[IBIS Ver]   4.1
[File Name]   tms570ls31x_21x_revc_pge_b.ibs
[File Rev]   1.0
[Date]   Tue Sep 17 07:21:23 2013
[Source]   Texas Instruments, Inc.
[Notes]   Revision History:
   1.0: initial release, 09/17/2013
   THIS IS RELEASE 1.0,THE CONTENTS ARE SUBJECT TO
   CHANGE WITHOUT PRIOR NOTICE,IF NECESSARY.
[Disclaimer] Please be aware that in the absence of a written agreement
   Texas Instruments(TI) assumes no liability for:
   (1) The accuracy of the IBIS models provided to your company
   (2) The proper functioning of these Models in your design
   or for any resulting applications;or
   (3) Infringement of patents,copyrights or intellectual
   property rights resulting from your use of these models.
   TI provides IBIS Models as a service to our customers and
   therefore reserves the right to limit distribution of the
   Models.
[Copyright]   Property of Texas Instruments Incorporated.
   Unauthorised reproduction and/or distribution is strictly.
   prohibited.
   This product is protected under copyright law and trade
   secret law as an unpublished work.
   Created 2013,(C) Copyright 2013-2014,
   Texas Instruments Incorporated., All Rights Reserved.
   These commodities are under the U.S. Government
   distribution license control.As such,they are not to be
   re-exported without the prior approval of the
   U.S. Department of Commerce.
[Component]   TMS570LS31x/21x_REVC_PGE_B
[Manufacturer]   Texas Instruments
[Package]
 | variable   typ   min   max
R_pkg   179.763m   7.91949m   216.493m
L_pkg   7.02661nH   2.0891nH   7.71072nH
C_pkg   0.955318pF   0.771641pF   6.68767pF
[Pin]	signal_name	model_name	R_pin	L_pin	C_pin
1	FRAYTX2	OQ0112FT	201.684m	7.04026nH	0.937901pF
2	FRAYRX2	IQ0442FT_40P60P	200.916m	7.42774nH	1.06436pF
3	MIBSPI3NCS[3]	BQ0210FT	198.584m	7.59867nH	1.05403pF
4	MIBSPI3NCS[2]	BQ0210FT	195.911m	7.63854nH	1.03198pF
5	FRAYTXEN2	OQ0112FT	195.321m	7.65814nH	1.00344pF
6	NHET1[11]	BQ0210FT	195.924m	7.67408nH	0.970612pF
|7	FLTP1	BAFTHRU15VFT	196.228m	7.64822nH	0.953678pF
|8	FLTP2	BAFTHRU8VFT	196.899m	7.58856nH	0.936175pF
9	GIOA[2]	BQ0215FT	200.797m	7.59854nH	0.910668pF
|10	VCCIO	VDDS33TF1_60UM	204.628m	7.57516nH	0.908233pF
|11	VSS	VSS00T2_60UM	203.393m	7.46268nH	0.896311pF
12	CAN3RX	BQ0210FT	204.531m	7.41325nH	0.865383pF
13	CAN3TX	BQ0210FT	212.37m	7.50397nH	0.859888pF
14	GIOA[5]	BQ0210FT	213.785m	7.48678nH	0.855034pF
15	NHET1[22]	BQ0215FT	213.017m	7.33523nH	0.854962pF
16	GIOA[6]	BQ0210FT	211.155m	7.25549nH	0.844253pF
|17	VCC	VDD12T1_100UM	120.798m	6.70564nH	0.867718pF
|18	OSCIN	IOSCHF33FTHY_NI	214.999m	7.2584nH	0.815084pF
|19	KELVIN_GND	VSS00T2_60UM	213.472m	7.23357nH	0.828091pF
|20	OSCOUT	OOSCHF33FT	209.627m	7.16687nH	0.835423pF
|21	VSS	VSS00T2_60UM	206.908m	7.15454nH	0.828833pF
22	GIOA[7]	BQ0210FT	207.016m	7.17268nH	0.825821pF
23	NHET1[01]	BQ0215FT	205.654m	7.15804nH	0.858767pF
24	NHET1[03]	BQ0215FT	202.592m	7.0987nH	0.878742pF
25	NHET1[0]	BQ0215FT	201.398m	7.17984nH	0.889476pF
|26	VCCIO	VDDS33TF1_60UM	116.258m	6.76964nH	0.963387pF
|27	VSS	VSS00T2_60UM	198.771m	7.34545nH	0.926279pF
|28	VSS	VSS00T2_60UM	198.014m	7.38253nH	0.949683pF
|29	VCC	VDD12T1_100UM	116.537m	6.9325nH	1.02223pF
30	NHET1[02]	BQ0215FT	198.729m	7.45545nH	0.966564pF
31	NHET1[05]	BQ0215FT	198.508m	7.51746nH	0.97276pF
32	MIBSPI5NCS[0]	BQ0210FT	198.713m	7.58776nH	1.00435pF
33	NHET1[07]	BQ0215FT	198.824m	7.63516nH	1.03075pF
34	TEST	BQ0213FT	202.469m	7.64935nH	1.04432pF
35	NHET1[09]	BQ0215FT	198.884m	7.46111nH	1.04914pF
36	NHET1[04]	BQ0210FT	201.493m	7.12235nH	0.932251pF
37	MIBSPI3NCS[1]	BQ0215FT	189.818m	6.90291nH	0.941411pF
38	NHET1[06]	BQ0210FT	181.261m	7.14802nH	1.05899pF
39	NHET1[13]	BQ0210FT	181.614m	7.41222nH	1.03625pF
40	MIBSPI1NCS[2]	BQ0215FT	174.499m	7.33051nH	1.01977pF
41	NHET1[15]	BQ0210FT	168.874m	7.24167nH	0.998916pF
|42	VCCIO	VDDS33TF1_60UM	164.766m	7.11249nH	0.963348pF
|43	VSS	VSS00T2_60UM	161.622m	6.97546nH	0.946437pF
|44	VSS	VSS00T2_60UM	159.787m	6.88564nH	0.937131pF
|45	VCC	VDD12T1_100UM	75.8295m	6.24953nH	0.974078pF
46	nPORRST	IQ0087FT	162.699m	6.8213nH	0.87771pF
|47	VSS	VSS00T2_60UM	161.89m	6.69562nH	0.870364pF
|48	VCC	VDD12T1_100UM	97.1908m	6.22797nH	0.900575pF
|49	VCC	VDD12T1_100UM	96.9924m	6.13153nH	0.88635pF
|50	VSS	VSS00T2_60UM	164.702m	6.51157nH	0.826317pF
51	MIBSPI3SOMI	BQ0211FT	166.102m	6.43655nH	0.804429pF
52	MIBSPI3SIMO	BQ0211FT	167.111m	6.3794nH	0.795778pF
53	MIBSPI3CLK	BQ0211FT	169.065m	6.34914nH	0.786551pF
54	MIBSPI3NENA	BQ0210FT	171.864m	6.3567nH	0.784271pF
55	MIBSPI3NCS[0]	BQ0210FT	174.472m	6.49861nH	0.788938pF
|56	VSS	VSS00T2_60UM	174.866m	6.48726nH	0.784451pF
|57	VCC	VDD12T1_100UM	76.8843m	5.8157nH	0.84495pF
|58	AD1IN[16]_AD2IN[0]	IQ0444FT5	167.871m	6.39938nH	0.7931pF
|59	AD1IN[17]_AD2IN[01]	IQ0444FT5	165.448m	6.40474nH	0.816553pF
|60	AD1IN[0]	IQ0078FT5	163.468m	6.43102nH	0.836345pF
|61	AD1IN[07]	IQ0078FT5	162.275m	6.47546nH	0.851244pF
|62	AD1IN[18]_AD2IN[02]	IQ0444FT5	161.555m	6.56596nH	0.859126pF
|63	AD1IN[19]_AD2IN[03]	IQ0444FT5	161.432m	6.67329nH	0.869256pF
|64	AD1IN[20]_AD2IN[04]	IQ0444FT5	161.381m	6.70182nH	0.90007pF
|65	AD1IN[21]_AD2IN[05]	IQ0444FT5	161.995m	6.77747nH	0.921382pF
|66	ADREFHI	BAFTHRU50FT	162.542m	6.90485nH	0.933116pF
|67	ADREFLO	BAFTHRU50FT	164.993m	7.01966nH	0.953953pF
|68	VSSAD	VSSA00T2_100UM	167.891m	7.07177nH	0.987652pF
|69	VCCAD	VDDA50TF2	171.939m	7.12571nH	1.0092pF
|70	AD1IN[09]_AD2IN[09]	IQ0444FT5	176.774m	7.19031nH	1.02717pF
|71	AD1IN[01]	IQ0078FT5	182.269m	7.07161nH	1.05417pF
|72	AD1IN[10]_AD2IN[10]	IQ0444FT5	188.41m	6.88307nH	0.930632pF
|73	AD1IN[02]	IQ0078FT5	199.512m	7.07604nH	0.937836pF
|74	AD1IN[03]	IQ0078FT5	196.43m	7.45714nH	1.06151pF
|75	AD1IN[11]_AD2IN[11]	IQ0444FT5	195.408m	7.65087nH	1.04087pF
|76	AD1IN[04]	IQ0078FT5	194.285m	7.71072nH	1.02379pF
|77	AD1IN[12]_AD2IN[12]	IQ0444FT5	194.295m	7.68045nH	1.00758pF
|78	AD1IN[05]	IQ0078FT5	195.169m	7.65467nH	0.97891pF
|79	AD1IN[13]_AD2IN[13]	IQ0444FT5	195.708m	7.58317nH	0.966122pF
|80	AD1IN[06]	IQ0078FT5	198.156m	7.53735nH	0.95599pF
|81	AD1IN[22]_AD2IN[06]	IQ0444FT5	199.148m	7.54285nH	0.92948pF
|82	AD1IN[14]_AD2IN[14]	IQ0444FT5	201.452m	7.53971nH	0.90262pF
|83	AD1IN[08]_AD2IN[08]	IQ0444FT5	204.034m	7.4573nH	0.891661pF
|84	AD1IN[23]_AD2IN[07]	IQ0444FT5	205.119m	7.4742nH	0.883899pF
|85	AD1IN[15]_AD2IN[15]	IQ0444FT5	206.638m	7.35868nH	0.864379pF
86	AD1EVT	BQ0210FT	205.68m	7.30192nH	0.836559pF
|87	VCC	VDD12T1_100UM	88.0539m	6.42383nH	0.922308pF
|88	VSS	VSS00T2_60UM	205.44m	7.16036nH	0.846531pF
89	CAN1TX	BQ0210FT	207.947m	7.16054nH	0.837647pF
90	CAN1RX	BQ0210FT	211.017m	7.16768nH	0.82523pF
91	NHET1[24]	BQ0210FT	212.306m	7.15051nH	0.826669pF
92	NHET1[26]	BQ0210FT	213.491m	7.22891nH	0.844168pF
93	MIBSPI1SIMO	BQ0211FT	215.474m	7.31019nH	0.845545pF
94	MIBSPI1SOMI	BQ0211FT	214.506m	7.3229nH	0.83827pF
95	MIBSPI1CLK	BQ0211FT	213.809m	7.40217nH	0.868381pF
96	MIBSPI1NENA	BQ0210FT	216.493m	7.50172nH	0.884186pF
97	MIBSPI5NENA	BQ0210FT	210.996m	7.42558nH	0.870334pF
98	MIBSPI5SOMI[0]	BQ0212FT	207.913m	7.31239nH	0.881672pF
99	MIBSPI5SIMO[0]	BQ0212FT	206.103m	7.33234nH	0.903194pF
100	MIBSPI5CLK	BQ0212FT	206.76m	7.43485nH	0.929874pF
|101	VCC	VDD12T1_100UM	199.781m	7.44261nH	0.938448pF
|102	VSS	VSS00T2_60UM	199.165m	7.56763nH	0.948344pF
|103	VSS	VSS00T2_60UM	197.046m	7.56124nH	0.976045pF
|104	VCCIO	VDDS33TF1_60UM	197.927m	7.57833nH	1.00913pF
105	MIBSPI1NCS[0]	BQ0215FT	196.658m	7.59451nH	1.02357pF
106	NHET1[08]	BQ0215FT	199.189m	7.59472nH	1.0449pF
107	NHET1[28]	BQ0215FT	198.581m	7.39713nH	1.04993pF
108	TMS	BQ0192FT	199.808m	7.05039nH	0.92717pF
109	nTRST	IQ0087FT	189.351m	6.93314nH	0.941519pF
110	TDI	BQ0192FT	180.833m	7.18053nH	1.06865pF
111	TDO	BQ0192FT	174.6m	7.30146nH	1.04099pF
112	TCK	IQ0079FT	168.129m	7.20332nH	1.0074pF
113	RTCK	OQ0112FT	164.996m	7.10969nH	0.971868pF
|114	VCC	VDD12T1_100UM	183.392m	7.38873nH	0.965351pF
|115	VSS	VSS00T2_60UM	178.077m	7.27224nH	0.953382pF
116	nRST	BQ0414FT	176.952m	7.2215nH	0.937805pF
117	nERROR	BQ0212FT	174.143m	7.11039nH	0.912062pF
118	NHET1[10]	BQ0215FT	174.219m	6.97097nH	0.889169pF
119	ECLK	BQ0215FT	170.748m	6.83875nH	0.875206pF
|120	VCCIO	VDDS33TF1_60UM	169.236m	6.73321nH	0.861787pF
|121	VSS	VSS00T2_60UM	166.709m	6.63449nH	0.840897pF
|122	VSS	VSS00T2_60UM	169.916m	6.72922nH	0.81904pF
|123	VCC	VDD12T1_100UM	99.72m	6.24773nH	0.842834pF
124	NHET1[12]	BQ0210FT	174.231m	6.61843nH	0.792641pF
125	NHET1[14]	BQ0215FT	173.472m	6.52561nH	0.783236pF
126	FRAYRX1	IQ0442FT_40P60P	173.246m	6.47199nH	0.771641pF
127	NHET1[30]	BQ0215FT	173.833m	6.46115nH	0.771688pF
128	CAN2TX	BQ0210FT	170.744m	6.41525nH	0.773058pF
129	CAN2RX	BQ0210FT	173.471m	6.45308nH	0.801657pF
130	MIBSPI1NCS[1]	BQ0215FT	169.083m	6.38503nH	0.815094pF
131	LINRX	BQ0210FT	166.559m	6.35471nH	0.824822pF
132	LINTX	BQ0210FT	163.671m	6.38226nH	0.836538pF
133	FRAYTX1	OQ0112FT	162.88m	6.42987nH	0.839891pF
|134	VCCP	VDDFT33TF	97.1337m	6.10946nH	0.895144pF
|135	VSS	VSS00T2_60UM	160.618m	6.63246nH	0.877099pF
|136	VCCIO	VDDS33TF1_60UM	159.375m	6.64065nH	0.908634pF
|137	VCC	VDD12T1_100UM	159.405m	6.687nH	0.928827pF
|138	VSS	VSS00T2_60UM	160.655m	6.80407nH	0.940362pF
139	NHET1[16]	BQ0210FT	163.282m	6.89936nH	0.962829pF
140	NHET1[18]	BQ0210FT	166.657m	6.95055nH	0.998875pF
141	NHET1[20]	BQ0210FT	171.862m	7.00459nH	1.01785pF
142	FRAYTXEN1	OQ0112FT	178.736m	7.09847nH	1.03593pF
|143	VCC	VDD12T1_100UM	181.802m	7.01727nH	1.05637pF
|144	VSS	VSS00T2_60UM	189.553m	6.84899nH	0.943956pF
[Model Selector] BQ0192FT
BQ0192FT_PZ_3P3  Cell operated at 3.3(nom)
|BQ0192FT_PZ_3P3; PUPD_OFF
BQ0192FT_PU_3P3  Cell operated at 3.3(nom)
|BQ0192FT_PU_3P3; PULLUP_ON
BQ0192FT_PD_3P3  Cell operated at 3.3(nom)
|BQ0192FT_PD_3P3; PULLDOWN_ON
[Model Selector] BQ0210FT
BQ0210FT_PZ_3P3  Cell operated at 3.3(nom)
|BQ0210FT_PZ_3P3; PUPD_OFF
BQ0210FT_PU_3P3  Cell operated at 3.3(nom)
|BQ0210FT_PU_3P3; PULLUP_ON
BQ0210FT_PD_3P3  Cell operated at 3.3(nom)
|BQ0210FT_PD_3P3; PULLDOWN_ON
[Model Selector] BQ0211FT
BQ0211FT_PZ_3P3  Cell operated at 3.3(nom)
|BQ0211FT_PZ_3P3; PUPD_OFF
BQ0211FT_PU_3P3  Cell operated at 3.3(nom)
|BQ0211FT_PU_3P3; PULLUP_ON
BQ0211FT_PD_3P3  Cell operated at 3.3(nom)
|BQ0211FT_PD_3P3; PULLDOWN_ON
[Model Selector] BQ0212FT
BQ0212FT_PZ_3P3  Cell operated at 3.3(nom)
|BQ0212FT_PZ_3P3; PUPD_OFF
BQ0212FT_PU_3P3  Cell operated at 3.3(nom)
|BQ0212FT_PU_3P3; PULLUP_ON
BQ0212FT_PD_3P3  Cell operated at 3.3(nom)
|BQ0212FT_PD_3P3; PULLDOWN_ON
[Model Selector] BQ0213FT
BQ0213FT_PZ_3P3  Cell operated at 3.3(nom)
|BQ0213FT_PZ_3P3; PULLDOWN_OFF
BQ0213FT_PD_3P3  Cell operated at 3.3(nom)
|BQ0213FT_PD_3P3; PULLDOWN_ON
[Model Selector] BQ0215FT
BQ0215FT_PZ_3P3  Cell operated at 3.3(nom)
|BQ0215FT_PZ_3P3; PUPD_OFF
BQ0215FT_PU_3P3  Cell operated at 3.3(nom)
|BQ0215FT_PU_3P3; PULLUP_ON
BQ0215FT_PD_3P3  Cell operated at 3.3(nom)
|BQ0215FT_PD_3P3; PULLDOWN_ON
[Model Selector] BQ0414FT
BQ0414FT_PZ_3P3  Cell operated at 3.3(nom)
|BQ0414FT_PZ_3P3; PUPD_OFF
BQ0414FT_PU_3P3  Cell operated at 3.3(nom)
|BQ0414FT_PU_3P3; PULLUP_ON
BQ0414FT_PD_3P3  Cell operated at 3.3(nom)
|BQ0414FT_PD_3P3; PULLDOWN_ON
[Model Selector] IQ0079FT
IQ0079FT_PZ_3P3  Cell operated at 3.3(nom)
|IQ0079FT_PZ_3P3; PUPD_OFF
IQ0079FT_PU_3P3  Cell operated at 3.3(nom)
|IQ0079FT_PU_3P3; PULLUP_ON
IQ0079FT_PD_3P3  Cell operated at 3.3(nom)
|IQ0079FT_PD_3P3; PULLDOWN_ON
[Model Selector] IQ0087FT
IQ0087FT_PZ_3P3  Cell operated at 3.3(nom)
|IQ0087FT_PZ_3P3; PULLDOWN_OFF
IQ0087FT_PD_3P3  Cell operated at 3.3(nom)
|IQ0087FT_PD_3P3; PULLDOWN_ON
[Model Selector] IQ0442FT_40P60P
0442FT_40P60P_PZ_3P3  Cell operated at 3.3(nom)
|IQ0442FT_40P60P_PZ_3P3; PUPD_OFF
2FT_40P60P_PU_3P3  Cell operated at 3.3(nom)
|IQ0442FT_40P60P_PU_3P3; PULLUP_ON
2FT_40P60P_PD_3P3  Cell operated at 3.3(nom)
| Models and submodels in the file (29): BQ0192FT_PZ_3P3 (I/O), BQ0192FT_PU_3P3 (I/O), BQ0192FT_PD_3P3 (I/O), BQ0210FT_PZ_3P3 (I/O), BQ0210FT_PU_3P3 (I/O), BQ0210FT_PD_3P3 (I/O), BQ0211FT_PZ_3P3 (I/O), BQ0211FT_PU_3P3 (I/O), BQ0211FT_PD_3P3 (I/O), BQ0212FT_PZ_3P3 (I/O), BQ0212FT_PU_3P3 (I/O), BQ0212FT_PD_3P3 (I/O), BQ0213FT_PZ_3P3 (I/O), BQ0213FT_PD_3P3 (I/O), BQ0215FT_PZ_3P3 (I/O), BQ0215FT_PU_3P3 (I/O), BQ0215FT_PD_3P3 (I/O), BQ0414FT_PZ_3P3 (I/O), BQ0414FT_PU_3P3 (I/O), BQ0414FT_PD_3P3 (I/O), IQ0079FT_PZ_3P3 (Input), IQ0079FT_PU_3P3 (Input), IQ0079FT_PD_3P3 (Input), IQ0087FT_PZ_3P3 (Input), IQ0087FT_PD_3P3 (Input), 0442FT_40P60P_PZ_3P3 (Input), 2FT_40P60P_PU_3P3 (Input), 2FT_40P60P_PD_3P3 (Input), OQ0112FT (3-state)
